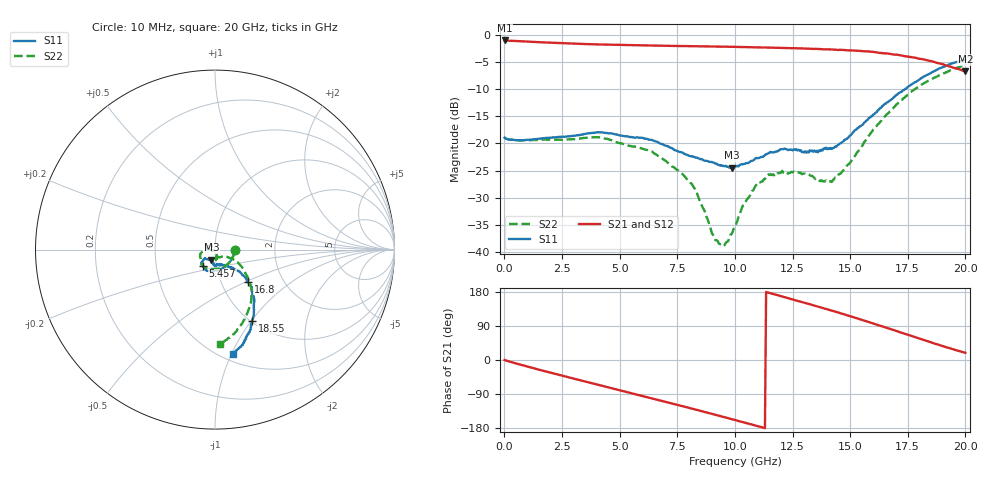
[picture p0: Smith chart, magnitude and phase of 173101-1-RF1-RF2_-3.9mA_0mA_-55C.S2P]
!  2-Port S-parameters saved by WinCal
! VAR MeasName=S-Parameters (CALIBRATED_DATA) read from VNA (N5242A)
! VAR MeasDate=2017-7-20 10:21:45
! VAR NAME=173101-1-RF1-RF2_-3.9mA_0mA_-55C
! VAR FILENAME=173101-1-RF1-RF2_-3.9mA_0mA_-55C.S2P
! VAR DATE=2017-7-20 10:21:45
! VAR PHYS_PORTS=1,2
# Hz S DB R 50
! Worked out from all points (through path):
!   401 points, 10 MHz to 20 GHz, reference 50 ohm
!   highest |S21| = -1.08 dB at 10 MHz (marker M1); lowest = -6.7 dB at 20 GHz (marker M2)
!   group delay of S21, straight-line fit = 46.7 ps
!   lowest |S11| = -24.5 dB at 9.855 GHz (marker M3), VSWR 1.13, Z = 47.7 - j5.38 ohm
!   |S11| at or under -10 dB: start of sweep to 17.39 GHz
!   |S22| runs from -38.9 to -5.6 dB; largest |S21 - S12| = 0.0072
!   S11 on the Smith chart (normalised r, x): 10 MHz: 1.25, -0.01; 5.457 GHz: 0.86, -0.16; 16.8 GHz: 1.34, -0.51; 18.55 GHz: 1.01, -1.02; 20 GHz: 0.57, -1.01
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1e7  -18.95 -2.4  -1.08 -0.0  -1.08 -0.1  -18.91 -2.1
1.50925e9  -19.14 -57.1  -1.40 -25.7  -1.41 -25.7  -19.35 -59.8
3.358325e9  -18.38 -98.8  -1.71 -54.5  -1.72 -54.5  -19.04 -108.7
4.157925e9  -17.97 -111.7  -1.82 -66.7  -1.83 -66.7  -18.91 -126.1
5.457275e9  -18.85 -125.3  -1.93 -86.6  -1.94 -86.5  -20.47 -147.6
6.70665e9  -19.90 -136.3  -2.02 -106.0  -2.02 -105.9  -22.40 -168.3
8.2059e9  -22.47 -139.0  -2.14 -129.4  -2.15 -129.5  -28.02 174.5
9.255375e9  -23.90 -119.5  -2.19 -146.2  -2.19 -146.3  -37.93 -141.6
9.555225e9  -24.21 -114.4  -2.22 -151.1  -2.23 -151.1  -38.68 -112.6
9.855075e9  -24.48 -109.8  -2.24 -155.9  -2.25 -156.0  -36.68 -93.9
1.0005e10  -24.26 -109.2  -2.26 -158.4  -2.27 -158.5  -35.25 -85.1
1.04048e10  -23.76 -102.8  -2.29 -164.9  -2.30 -165.0  -31.28 -75.1
1.085458e10  -22.90 -99.7  -2.34 -172.3  -2.36 -172.4  -28.08 -73.6
1.145428e10  -21.80 -97.3  -2.39 177.8  -2.41 177.8  -25.70 -79.3
1.255372e10  -21.11 -86.7  -2.50 159.1  -2.52 159.2  -25.16 -85.7
1.335332e10  -21.29 -80.9  -2.61 145.2  -2.59 145.2  -25.96 -83.0
1.430285e10  -20.83 -66.3  -2.77 128.3  -2.78 128.3  -26.55 -63.4
1.555222e10  -16.53 -45.0  -3.06 105.1  -3.07 104.9  -20.28 -29.2
1.670165e10  -12.15 -43.3  -3.52 82.6  -3.58 82.2  -14.22 -35.1
1.68016e10  -11.86 -44.1  -3.62 80.6  -3.62 80.8  -13.78 -36.7
1.855072e10  -6.92 -62.5  -4.90 45.7  -4.99 45.7  -8.16 -62.0
2e10  -4.57 -80.2  -6.73 19.1  -6.79 19.6  -5.58 -86.7
